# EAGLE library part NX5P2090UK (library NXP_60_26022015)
Logic controlled high-side power switch The NX5P2090 is an advanced power switch for USB OTG applications. It includes under-voltage and over-voltage lockout, over-current, over-temperature, reverse bias and in-rush current protection circuits. These are designed to automatically isolate a VBUS OTG voltage source from a VBUS interface pin when a fault occurs. The device features two power switch terminals, one input (VINT) and one output (VBUS); a current limit input (ILIM) for defining the over-current and in-rush current limit; a voltage detect output (VDET) to monitor the voltage level on VBUS; an open-drain fault output (FAULT) to indicate when a fault condition has occurred and an enable input (EN) to control the state of the switch. When EN is set LOW the device enters a low-power mode, disabling all protection circuits accept the under-voltage lockout. The low-power mode can be entered at anytime unless the over temperature protection circuit has been triggered. Designed for operation from 3 V to 5.5 V, it is used in power domain isolation applications to protect from out of range operation. The enable input includes integrated logic level translation making the device compatible with lower voltage processors and controllers AAL Eindhoven MK
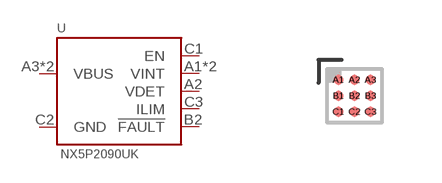
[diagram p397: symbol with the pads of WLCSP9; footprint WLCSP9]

Designator prefix U

## NX5P2090UK  [WLCSP9]
A1  VINT  pwr
A2  VDET  out
A3  VBUS  pwr
B1  VINT  pwr
B2  !FAULT  out
B3  VBUS  pwr
C1  EN  in
C2  GND  pwr
C3  ILIM  in

## Footprint WLCSP9 (pad centres in mm)
smd 0.25 x 0.25: A1 -0.4,0.4; A2 0,0.4; A3 0.4,0.4; B1 -0.4,0; B2 0,0; B3 0.4,0; C1 -0.4,-0.4; C2 0,-0.4; C3 0.4,-0.4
